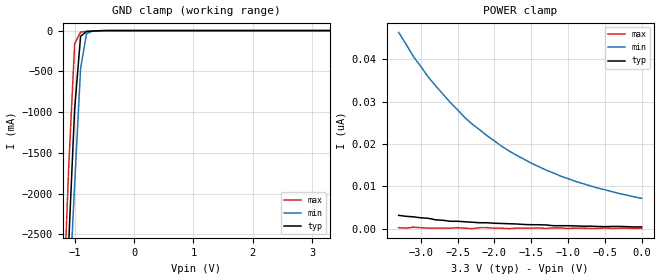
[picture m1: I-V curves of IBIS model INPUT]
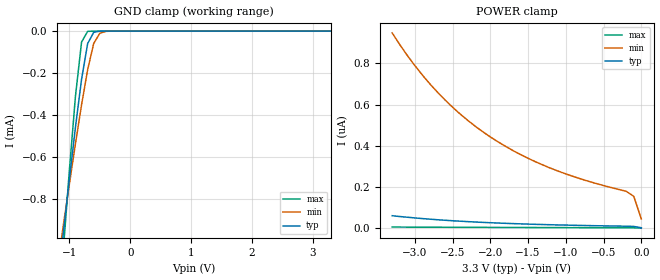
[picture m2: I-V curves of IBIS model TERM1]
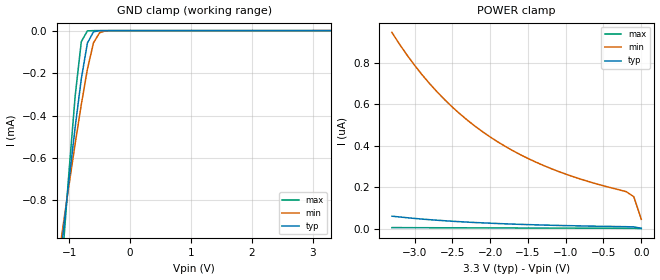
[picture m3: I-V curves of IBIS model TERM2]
|   DIODES INCORPORATED
|   IBIS Model of PI3DBS3224
|   Product Family: 3DBS
|   TQFN (ZNA) Package
[IBIS Ver] 4.0
[Comment char] |_char
[File Name] pi3dbs3224_zf_reva.ibs
[File Rev] 1.0
[Source] File originated at Diodes Incorporated.
[Date] 02/15/19
[Disclaimer] (C) Copyright DIODES INCORPORATED
   All rights reserved
  Diodes Incorporated hereby grants the user of
  this IBIS model a non-exclusive, nontransferable license to
  use this IBIS model under the following terms.
  This IBIS model is provided on an "AS IS" basis and Diodes
  makes absolutely no warranty with respect to the information
  contained herein. DIODES DISCLAIMS AND CUSTOMER WAIVES ALL
  WARRANTIES, EXPRESSED OR IMPLIED, INCLUDING WARRANTIES OF
  MERCHANTABILITY OR FITNESS FOR A PARTICULAR PURPOSE. The
  entire risk as to quality and performance is with the customer.
  Accordingly, in no event shall the company be liable for any
  damages, whether in contract or tort, including any lost
  profits or other incidental, consequential, exemplary, or
  punitive damages arising out of the use or application of the
  IBIS model provided in this package. Further, Diodes reserves
  the right to make changes without notice to any product herein
  to improve reliability, function, or design. Diodes does not
  convey any license under patent rights or any other intellectual
  property rights, including those of third parties.
  The user is granted this license only to use the IBIS model
  and is not granted rights to sell, load, rent, lease or license
  the IBIS model in whole or in part, or in modified form to anyone
  other than user. User may modify the IBIS model to suit its specific
  application but rights to derivative works and such modifications
  shall belong to Diodes.
  Diodes is not obligated to provide maintenance or support
  for the licensed IBIS model.
  Contact Diodes at ATTN: APPLICATION ENGINEERING / IBIS MODELS
  1545 Barber Lane Milpitas, CA 95035 USA.
[Component] PI3DBS3224
[Manufacturer] Diodes Incorporated.
[Package]
| variable   typ   min   max
R_pkg   0.02106ohm   0.01714ohm   0.02498ohm
L_pkg   1.00200nH   0.81800nH   1.18600nH
C_pkg   0.20050pF   0.19950pF   0.20550pF
[Pin] signal_name   model_name   R_pin   L_pin   C_pin
1   INA+   TERM1   0.02498   1.18600nH   0.20550pF
2   INA-   TERM1   0.02106   1.00200nH   0.20050pF
3   INB+   TERM1   0.01714   0.81800nH   0.19950pF
4   INB-   TERM1   0.01714   0.81800nH   0.19950pF
5   GND   GND   0.02106   1.00200nH   0.20050pF
6   OUTB1+   TERM2   0.02498   1.18600nH   0.20550pF
7   OUTB1-   TERM2   0.02498   1.18600nH   0.20550pF
8   OUTB0+   TERM2   0.02086   0.98900nH   0.20000pF
9   OUTB0-   TERM2   0.02086   0.98900nH   0.20000pF
10   ENB   INPUT   0.02498   1.18600nH   0.20550pF
11   SBO   INPUT   0.02498   1.18600nH   0.20550pF
12   SBI   INPUT   0.02106   1.00200nH   0.20050pF
13   VCC   POWER   0.01714   0.81800nH   0.19950pF
14   SAI   INPUT   0.01714   0.81800nH   0.19950pF
15   SAO   INPUT   0.02106   1.00200nH   0.20050pF
16   ENA   INPUT   0.02498   1.18600nH   0.20550pF
17   OUTA0-   TERM2   0.02498   1.18600nH   0.20550pF
18   OUTA0+   TERM2   0.02086   0.98900nH   0.20000pF
19   OUTA1-   TERM2   0.02086   0.98900nH   0.20000pF
20   OUTA1+   TERM2   0.02498   1.18600nH   0.20550pF
[Series Switch Groups]
| Function Group States
Off 1 2 3 4 5 6 7 8 /
On 2 7 /
On 1 7 /
On 6 7 /
On 5 7 /
On 2 8 /
On 1 8 /
On 6 8 /
On 5 8 /
On 2 3 /
On 1 3 /
On 6 3 /
On 5 3 /
On 2 4 /
On 1 4 /
On 6 4 /
On 5 4 /
On 1 /
On 2 /
On 3 /
On 4 /
On 5 /
On 6 /
On 7 /
On 8 /
[Series_Pin_Mapping]   pin_2   model_name   function_table_group
1   6   SWITCH   1
2   7   SWITCH   1
1   8   SWITCH   2
2   9   SWITCH   2
1   18   SWITCH   3
2   17   SWITCH   3
1   20   SWITCH   4
2   19   SWITCH   4
3   6   SWITCH   5
4   7   SWITCH   5
3   8   SWITCH   6
4   9   SWITCH   6
3   18   SWITCH   7
4   17   SWITCH   7
3   20   SWITCH   8
4   19   SWITCH   8
[Diff pin] inv_pin vdiff tdelay_typ tdelay_min tdelay_max
1   2   NA   NA   NA   NA
3   4   NA   NA   NA   NA
6   7   NA   NA   NA   NA
8   9   NA   NA   NA   NA
18   17   NA   NA   NA   NA
20   19   NA   NA   NA   NA
|   Model SWITCH1
[Model] SWITCH
Model_type Series_switch
| variable   typ   min   max
C_comp   3.2613pF   3.1495pF   3.4096pF
[Voltage Range]   3.3000V   3.0000V   3.6000V
[GND Clamp Reference]   0.0000V   0.0000V   0.0000V
[POWER Clamp Reference]   3.3000V   3.0000V   3.6000V
[temperature range]   25   85   -40
[On]
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[OFF]
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| Models and submodels in the file (4): INPUT (Input), SWITCH (Series_switch), TERM1 (Terminator), TERM2 (Terminator)
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|   Model INPUT
[Model] INPUT
Model_type Input
Vinl = 800mV
Vinh = 2.00V
| variable   typ   min   max
C_comp   1.5862pF   1.5826pF   1.5899pF
[Voltage Range]   3.3000V   3.0000V   3.6000V
[GND Clamp Reference]   0.0000V   0.0000V   0.0000V
[POWER Clamp Reference]   3.3000V   3.0000V   3.6000V
[temperature range]   25   85   -40
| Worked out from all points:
|   GND clamp passes 1 mA (typ) near -0.53 V on its own axis
[GND Clamp]
| Voltage   I(typ)   I(min)   I(max)
-3.3V     -38.82A    -36.04A    -42.73A
-1.2V     -4.251A    -4.855A    -3.541A
-1.1V     -2.605A    -3.371A    -1.675A
-1V       -958.7mA   -1.886A    -162.6mA
-900mV    -70.22mA   -465.8mA   -17.88mA
-800mV    -11.61mA   -38.16mA   -10.5mA
-700mV    -5.86mA    -7.386mA   -5.372mA
3.3V      407.5pA    8.265nA    116.4pA
[POWER Clamp]
| Voltage   I(typ)   I(min)   I(max)
-3.3V     3.143nA    46.33nA    232.8pA
-3.1V     2.794nA    40.63nA    349.3pA
-2.9V     2.445nA    35.86nA    116.4pA
-2.6V     1.746nA    29.8nA     116.4pA
-2.4V     1.63nA     26.19nA    116.4pA
-2.3V     1.513nA    24.68nA    0A
-2.2V     1.397nA    23.34nA    232.8pA
-1.9V     1.222nA    19.44nA    116.4pA
-1.5V     931.3pA    15.48nA    116.4pA
-1.1V     698.5pA    12.4nA     174.6pA
-600mV    523.9pA    9.604nA    58.21pA
0V        407.5pA    7.16nA     58.21pA
|   Model TERM1
[Model] TERM1
Model_type Terminator
| variable   typ   min   max
C_comp   2.5796pF   2.5185pF   2.6532pF
[Voltage Range]   3.3000V   3.0000V   3.6000V
[GND Clamp Reference]   0.0000V   0.0000V   0.0000V
[POWER Clamp Reference]   3.3000V   3.0000V   3.6000V
[temperature range]   25   85   -40
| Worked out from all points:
|   GND clamp passes 1 mA (typ) near -1.11 V on its own axis
[GND Clamp]
| Voltage   I(typ)   I(min)   I(max)
-3.3V     -1.768A    -1.849A    -1.692A
-1.2V     -1.227mA   -1.133mA   -1.44mA
-1.1V     -963.1uA   -926.3uA   -1.045mA
-1V       -705.2uA   -728.2uA   -663.2uA
-900mV    -457uA     -535.4uA   -309.2uA
-800mV    -229.2uA   -351.1uA   -52.48uA
-700mV    -59.12uA   -183.6uA   -1.239uA
-600mV    -5.582uA   -58.15uA   -10.57nA
-500mV    -191.1nA   -10.09uA   -291pA
-400mV    -4.562nA   -983.4nA   -211pA
3.3V      2.91nA     188.9nA    349.2pA
[POWER Clamp]
| Voltage   I(typ)   I(min)   I(max)
-3.3V     61.35nA    947.7nA    6.403nA
-3.1V     54.02nA    838.8nA    6.054nA
-2.8V     44.59nA    700.4nA    5.588nA
-2.5V     36.9nA     587.5nA    5.239nA
-2.2V     30.85nA    495.3nA    5.006nA
-1.8V     24.45nA    398nA      4.424nA
-1.6V     21.89nA    357.9nA    4.249nA
-1.3V     18.57nA    306.7nA    3.9nA
-800mV    14.2nA     239.6nA    3.376nA
-200mV    10.48nA    179.6nA    2.794nA
-100mV    9.43nA     155.5nA    2.619nA
0V        2.91nA     45.87nA    989.5pA
|   Model TERM2
[Model] TERM2
Model_type Terminator
| variable   typ   min   max
C_comp   1.5466pF   1.4931pF   1.6172pF
[Voltage Range]   3.3000V   3.0000V   3.6000V
[GND Clamp Reference]   0.0000V   0.0000V   0.0000V
[POWER Clamp Reference]   3.3000V   3.0000V   3.6000V
[temperature range]   25   85   -40
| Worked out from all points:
|   GND clamp passes 1 mA (typ) near -1.12 V on its own axis
[GND Clamp]
| Voltage   I(typ)   I(min)   I(max)
-3.3V     -1.034A    -1.059A    -1.02A
-1.2V     -1.221mA   -1.127mA   -1.432mA
-1.1V     -958uA     -921.7uA   -1.039mA
-1V       -701uA     -724.3uA   -658.7uA
-900mV    -454uA     -532.2uA   -307uA
-800mV    -227.6uA   -348.6uA   -52.27uA
-700mV    -58.81uA   -182.2uA   -1.239uA
-600mV    -5.575uA   -57.73uA   -10.55nA
-500mV    -191nA     -10.05uA   -305.6pA
-400mV    -4.555nA   -981.2nA   -181.9pA
3.3V      2.619nA    188.7nA    174.6pA
[POWER Clamp]
| Voltage   I(typ)   I(min)   I(max)
-3.3V     61nA       947.3nA    5.821nA
-3.1V     53.55nA    838.3nA    5.588nA
-2.8V     44.01nA    700nA      5.239nA
-2.5V     36.44nA    587.1nA    4.889nA
-2.2V     30.38nA    495.1nA    4.657nA
-1.8V     24.04nA    397.6nA    4.075nA
-1.6V     21.48nA    357.6nA    3.9nA
-1.3V     18.22nA    306.5nA    3.609nA
-800mV    13.91nA    239.3nA    3.143nA
-200mV    10.25nA    179.2nA    2.503nA
-100mV    9.197nA    155.3nA    2.386nA
0V        2.619nA    45.69nA    756.7pA
